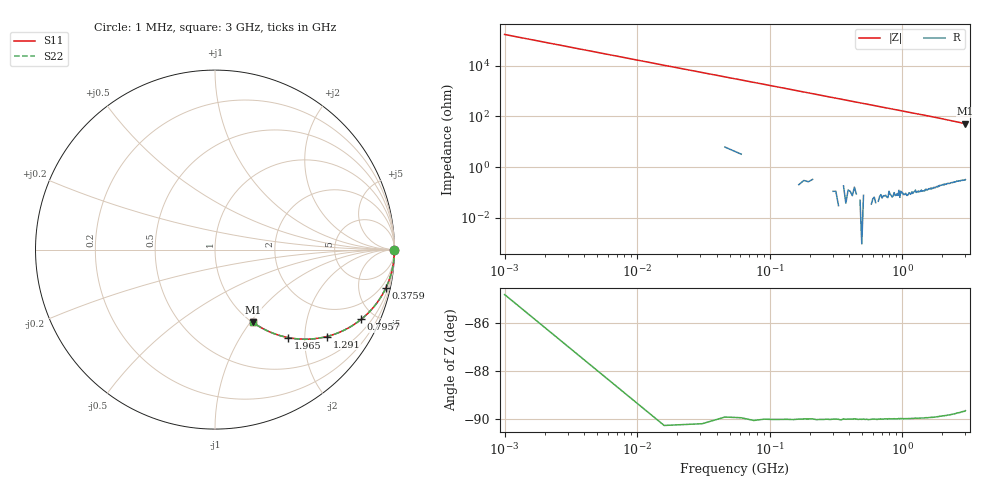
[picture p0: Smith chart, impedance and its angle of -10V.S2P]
!Keysight Technologies,E4991B,MY54301043,A.02.04
!Date: Thu Nov 16 21:16:53 2023
!Data:
!Freq	S11	S21	S12	S22
# Hz S MA R 50
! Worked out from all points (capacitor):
!   201 points, 1 MHz to 3 GHz, reference 50 ohm
!   read as one part in series: C = 948 fF near 15.99 MHz
!   lowest |Z| = 51.6 ohm at 3 GHz (marker M1)
!   S11 on the Smith chart (normalised r, x): 1 MHz: open; 375.9 MHz: 1.00, -8.93; 795.7 MHz: 1.00, -4.20; 1.291 GHz: 1.00, -2.57; 1.965 GHz: 1.00, -1.66; 3 GHz: 1.01, -1.03
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1000000  0.9999 -0.0  0.0005846 84.8  0.0005846 84.8  0.9999 -0.0
1.5995e7  1 -0.5  0.009572 89.7  0.009572 89.7  1 -0.5
3.099e7  0.9999 -1.1  0.01845 89.1  0.01845 89.1  0.9999 -1.1
4.5985e7  0.9996 -1.6  0.02736 88.3  0.02736 88.3  0.9996 -1.6
6.098e7  0.9993 -2.1  0.0363 87.9  0.0363 87.9  0.9993 -2.1
7.5975e7  0.999 -2.6  0.04523 87.5  0.04523 87.5  0.999 -2.6
1.05965e8  0.998 -3.6  0.06299 86.4  0.06299 86.4  0.998 -3.6
1.35955e8  0.9967 -4.6  0.08078 85.4  0.08078 85.4  0.9967 -4.6
1.8094e8  0.9942 -6.2  0.1072 83.8  0.1072 83.8  0.9942 -6.2
2.25925e8  0.9911 -7.7  0.1334 82.3  0.1334 82.3  0.9911 -7.7
2.7091e8  0.9872 -9.2  0.1593 80.8  0.1593 80.8  0.9872 -9.2
3.75875e8  0.9758 -12.6  0.2187 77.4  0.2187 77.4  0.9758 -12.6
5.1083e8  0.9565 -17.0  0.2916 73.0  0.2916 73.0  0.9565 -17.0
6.45785e8  0.933 -21.1  0.36 68.9  0.36 68.9  0.933 -21.1
7.95735e8  0.9028 -25.4  0.4297 64.5  0.4297 64.5  0.9028 -25.4
1.005665e9  0.8561 -31.1  0.5163 58.9  0.5163 58.9  0.8561 -31.1
1.29057e9  0.7891 -37.8  0.6136 52.1  0.6136 52.1  0.7891 -37.8
1.5005e9  0.74 -42.2  0.6717 47.7  0.6717 47.7  0.74 -42.2
1.965345e9  0.638 -50.2  0.7685 39.6  0.7685 39.6  0.638 -50.2
2.01033e9  0.6289 -50.9  0.7759 39.0  0.7759 39.0  0.6289 -50.9
2.505165e9  0.5359 -57.4  0.842 32.4  0.842 32.4  0.5359 -57.4
3e9  0.4571 -62.4  0.8865 27.2  0.8865 27.2  0.4571 -62.4
